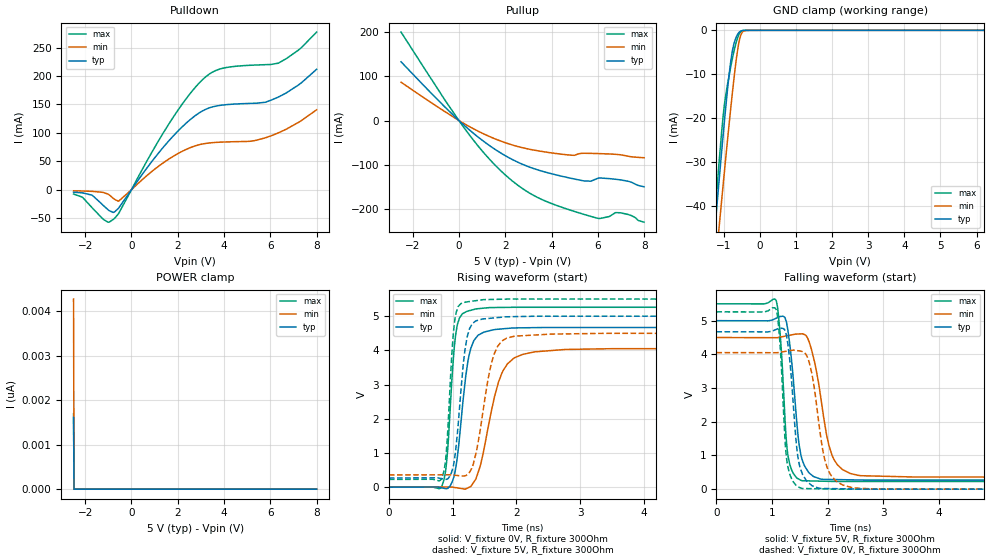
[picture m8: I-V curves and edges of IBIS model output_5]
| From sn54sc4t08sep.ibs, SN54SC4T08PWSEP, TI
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|   output_5p0 Model
[Model]   output_5
Model_type   3-state
Polarity   Non-Inverting
Vmeas = 2.5
Vref = 0
Cref = 2pF
Rref = 100000
|   typ   min   max
C_comp   5.7pF   5.6pF   6pF
[Voltage Range]   5   4.5   5.5
[Temperature Range]   25   125   -40
[Pullup Reference]   5   4.5   5.5
[Pulldown Reference]   0   0   0
[Power Clamp Reference]   5   4.5   5.5
[GND Clamp Reference]   0   0   0
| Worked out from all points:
|   slope of the pulldown table from 0 to 0.75 V, typ, clamps not added: 17.6 ohm
|   slope of the pullup table from 0 to 0.75 V, typ, clamps not added: 22 ohm
|   GND clamp passes 1 mA (typ) near -0.62 V on its own axis
|   falling waveform, V_fixture 5V, R_fixture 300Ohm: 20-80 % time 162ps typ, 266ps min, 113ps max; typ from 5 V to 0.269 V
|   rising waveform, V_fixture 0V, R_fixture 300Ohm: 20-80 % time 168ps typ, 297ps min, 112ps max; typ from 0 V to 4.67 V
|   rising waveform, V_fixture 5V, R_fixture 300Ohm: 20-80 % time 142ps typ, 228ps min, 98.1ps max; typ from 0.269 V to 5 V
|   falling waveform, V_fixture 0V, R_fixture 300Ohm: 20-80 % time 144ps typ, 223ps min, 105ps max; typ from 4.67 V to 0 V
[Pulldown]
|   Voltage   I(typ)   I(min)   I(max)
-2.5V     -4.172mA   -1.772mA   -7.441mA
-2.122V   -5.347mA   -2.105mA   -12.9mA
-1.702V   -9.4mA     -2.721mA   -31.36mA
-1.009V   -35.09mA   -7.698mA   -56.94mA
-788.5mV  -39.73mA   -14.85mA   -52.23mA
-557.5mV  -32.38mA   -20.14mA   -42.06mA
1.605V    85.59mA    53.79mA    115mA
3.075V    138.8mA    80.61mA    193.8mA
3.958V    149.1mA    83.96mA    213.8mA
5.28V     152.1mA    86.21mA    219.2mA
6.351V    163.2mA    100.1mA    222.7mA
8V        211.9mA    140.6mA    277.3mA
[GND Clamp]
|   Voltage   I(typ)   I(min)   I(max)
-2.5V     -170.7mA   -168.9mA   -187.4mA
-1.282V   -49.09mA   -58.54mA   -46.61mA
-1.24V    -45.04mA   -54.83mA   -42.02mA
-1.208V   -42.02mA   -52.06mA   -38.61mA
-1.125V   -34.05mA   -44.71mA   -29.82mA
-977.5mV  -20.62mA   -32.07mA   -16.86mA
-799mV    -6.847mA   -17.4mA    -8.124mA
-715mV    -3.091mA   -11.05mA   -4.817mA
-641.5mV  -1.357mA   -6.134mA   -2.454mA
-526mV    -161.3uA   -1.092mA   -287.1uA
-379mV    -1.459uA   -24.15uA   -792nA
8V        0A         0A         0A
[Pullup]
|   Voltage   I(typ)   I(min)   I(max)
-2.5V     133.2mA    86.84mA    200.6mA
-610mV    30.93mA    20.35mA    46.86mA
429.5mV   -20.16mA   -13.03mA   -31.05mA
1.406V    -59.92mA   -38.19mA   -92.51mA
2.341V    -89.31mA   -55.94mA   -138.5mA
3.517V    -113.7mA   -69.57mA   -177.5mA
4.84V     -131mA     -78.59mA   -203.7mA
5.197V    -134.8mA   -75.08mA   -209.6mA
5.7V      -137.5mA   -74.5mA    -217.5mA
6.068V    -130.3mA   -75.07mA   -222.2mA
6.971V    -134.5mA   -77.65mA   -209.3mA
8V        -150.3mA   -84.37mA   -230.6mA
[POWER Clamp]
|   Voltage   I(typ)   I(min)   I(max)
-2.5V     1.612nA    4.273nA    1.696nA
-2.479V   0A         0A         0A
-2.469V   0A         0A         0A
8V        0A         0A         0A
[Ramp]
R_load = 300
|   typ   min   max
dV/dt_r   2.80224/1.67743e-10   2.43143/2.93578e-10   3.15661/1.12098e-10
dV/dt_f   2.83886/1.60456e-10   2.48482/2.63354e-10   3.16355/1.12372e-10
[Falling Waveform]
V_fixture = 5V
V_fixture_min = 4.5V
V_fixture_max = 5.5V
R_fixture = 300Ohm
C_fixture = 0F
|   Time   V(typ)   V(min)   V(max)
0s        5V         4.5V       5.5V
1.069ns   5.069V     4.494V     5.607V
1.151ns   5.125V     4.514V     4.471V
1.28ns    4.755V     4.556V     1.06V
1.471ns   1.52V      4.605V     305.9mV
1.528ns   949.7mV    4.609V     255.3mV
1.708ns   424.1mV    4.146V     244.1mV
2.075ns   287.1mV    1.014V     230.2mV
2.546ns   272.9mV    409.8mV    227.6mV
15ns      268.5mV    358.6mV    227.4mV
[Rising Waveform]
V_fixture = 0V
V_fixture_min = 0V
V_fixture_max = 0V
R_fixture = 300Ohm
C_fixture = 0F
|   Time   V(typ)   V(min)   V(max)
0s        6.167uV    3.711uV    7.4uV
828.7ps   -20.01mV   3.89mV     25.7mV
903.9ps   -44.28mV   4.243mV    716.8mV
1.012ns   262.6mV    -2.778mV   3.796V
1.069ns   830.4mV    -20.09mV   4.712V
1.238ns   3.674V     -21.51mV   5.149V
1.359ns   4.352V     226mV      5.209V
1.773ns   4.628V     3.341V     5.255V
2.28ns    4.664V     3.954V     5.26V
15ns      4.67V      4.052V     5.261V
[Rising Waveform]
V_fixture = 5V
V_fixture_min = 4.5V
V_fixture_max = 5.5V
R_fixture = 300Ohm
C_fixture = 0F
|   Time   V(typ)   V(min)   V(max)
0s        268.5mV    358.6mV    227.4mV
831.1ps   249.9mV    361.4mV    272.2mV
899.6ps   228.7mV    361.6mV    1.02V
987.3ps   464mV      356.8mV    3.91V
1.03ns    842.7mV    349.1mV    4.839V
1.202ns   4.124V     338.1mV    5.412V
1.37ns    4.867V     1.032V     5.455V
1.644ns   4.948V     3.862V     5.49V
1.959ns   4.986V     4.41V      5.499V
15ns      5V         4.5V       5.5V
[Falling Waveform]
|Gnd
V_fixture = 0V
V_fixture_min = 0V
V_fixture_max = 0V
R_fixture = 300Ohm
C_fixture = 0F
|   Time   V(typ)   V(min)   V(max)
0s        4.67V      4.053V     5.261V
1.069ns   4.737V     4.049V     5.342V
1.144ns   4.774V     4.063V     4.266V
1.266ns   4.495V     4.095V     839.5mV
1.438ns   1.323V     4.113V     98.98mV
1.528ns   527.8mV    4.093V     23.78mV
1.686ns   145.5mV    3.641V     14.95mV
1.986ns   19.06mV    656.6mV    5.287mV
2.433ns   6.936mV    47.23mV    228.5uV
15ns      6.378uV    4.356uV    7.408uV
